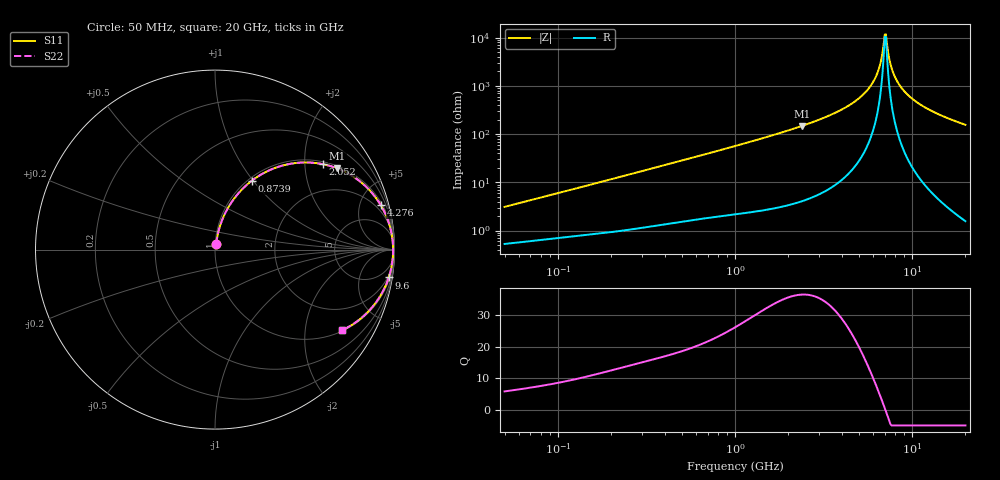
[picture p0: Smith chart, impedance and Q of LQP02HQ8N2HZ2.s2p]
!Murata Part Number: LQP02HQ8N2HZ2
!These Parameters are Measured in Series Mode Connection
!  o--[Z]--o
!Port1  Port2
!  o-------o
!Freq. Start=50[MHz] Stop=20[GHz], 401[Steps]
# Hz S RI R 50
!Freq.(Hz) S11(Real) S11(Imag) S21(Real) S21(Imag) S12(Real) S12(Imag) S22(Real) S22(Imag)
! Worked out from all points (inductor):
!   401 points, 50 MHz to 20 GHz, reference 50 ohm
!   read as one part in series: L = 9.62 nH near 51.52 MHz
!   highest Q = 36.5 at 2.384 GHz (marker M1), where L = 9.85 nH
!   self-resonance near 7.009 GHz
!   S11 on the Smith chart (normalised r, x): 50 MHz: 1.01, +0.06; 873.9 MHz: 1.04, +0.98; 2.052 GHz: 1.07, +2.46; 4.276 GHz: 1.28, +7.38; 9.6 GHz: 2, -12; 20 GHz: 1.03, -3.12
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5e7  0.00617 0.0302  0.9938 -0.0302  0.9938 -0.0302  0.00617 0.0302
1.364002e8  0.014 0.078  0.986 -0.078  0.986 -0.078  0.014 0.078
3.721004e8  0.054 0.1976  0.946 -0.1976  0.946 -0.1976  0.054 0.1976
8.738837e8  0.2048 0.3834  0.7952 -0.3834  0.7952 -0.3834  0.2048 0.3834
1e9  0.25 0.4143  0.75 -0.4143  0.75 -0.4143  0.25 0.4143
2.05233e9  0.5995 0.4762  0.4005 -0.4762  0.4005 -0.4762  0.5995 0.4762
2.383959e9  0.6807 0.4527  0.3193 -0.4527  0.3193 -0.4527  0.6807 0.4527
2.728004e9  0.7495 0.4197  0.2505 -0.4197  0.2505 -0.4197  0.7495 0.4197
4.275624e9  0.9237 0.2473  0.0763 -0.2473  0.0763 -0.2473  0.9237 0.2473
5.273168e9  0.9689 0.1472  0.0311 -0.1472  0.0311 -0.1472  0.9689 0.1472
6.034176e9  0.9854 0.0799  0.0146 -0.0799  0.0146 -0.0799  0.9854 0.0799
6.503449e9  0.9903 0.0419  0.00967 -0.0419  0.00967 -0.0419  0.9903 0.0419
6.905011e9  0.9922 0.0115  0.00783 -0.0115  0.00783 -0.0115  0.9922 0.0115
7.009217e9  0.9923 0.00385  0.00767 -0.00385  0.00767 -0.00385  0.9923 0.00385
7.222371e9  0.9923 -0.0114  0.0077 0.0114  0.0077 0.0114  0.9923 -0.0114
7.442007e9  0.9918 -0.0267  0.00821 0.0267  0.00821 0.0267  0.9918 -0.0267
7.784049e9  0.9901 -0.0495  0.00986 0.0495  0.00986 0.0495  0.9901 -0.0495
8.141811e9  0.9874 -0.0724  0.0126 0.0724  0.0126 0.0724  0.9874 -0.0724
8.774992e9  0.9805 -0.1102  0.0195 0.1102  0.0195 0.1102  0.9805 -0.1102
9.600142e9  0.9682 -0.1551  0.0318 0.1551  0.0318 0.1551  0.9682 -0.1551
1.295331e10  0.8952 -0.2965  0.1048 0.2965  0.1048 0.2965  0.8952 -0.2965
2e10  0.7067 -0.4503  0.2933 0.4503  0.2933 0.4503  0.7067 -0.4503
